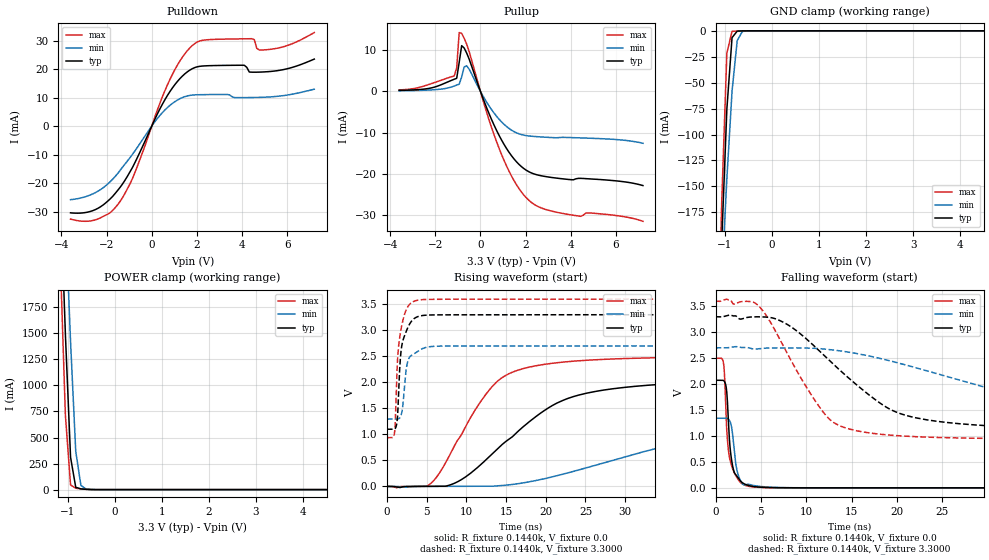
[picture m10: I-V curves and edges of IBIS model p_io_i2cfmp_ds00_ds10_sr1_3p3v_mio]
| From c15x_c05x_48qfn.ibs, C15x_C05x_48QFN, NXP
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[Model] p_io_i2cfmp_ds00_ds10_sr1_3p3v_mio
|   Model p_io_i2cfmp_ds00_ds10_sr1_3p3v_mio
| This model was characterised for following simulation conditions:
| External (pad) voltage:
|   - Typ: 3.3V,   - Min: 2.7V,   - Max: 3.6V
| Library cells for typ/min/max conditions are connected as defined below:
|  pad - External Pad
|  ipp_do_lv - Core Input
|  ipp_obe_lv - Output Buffer Enable
|  IOGC - NC
|  REFH3V3 - REFH3V3
|  REFL3V3 - REFL3V3
|  ZI - NC
|  abut_ncal_vddio[1] - vddio
|  abut_ncal_vddio[2] - vddio
|  abut_ncal_vddio[3] - vssio
|  abut_ncal_vddio[4] - vddio
|  abut_ncal_vddio[5] - vddio
|  abut_ncal_vddio[6] - vssio
|  abut_pcal_vddio[1] - vssio
|  abut_pcal_vddio[2] - vssio
|  abut_pcal_vddio[3] - vddio
|  abut_pcal_vddio[4] - vssio
|  abut_pcal_vddio[5] - vssio
|  abut_pcal_vddio[6] - vddio
|  ipp_do_1p8v - ipp_do_1p8v
|  ipp_dse_lv[0] - 0
|  ipp_dse_lv[1] - 0
|  ipp_eftd_lv - NC
|  ipp_ina_mux_vddio - NC
|  ipp_ina_mux_vddio[0] - NC
|  ipp_ina_mux_vddio[1] - NC
|  ipp_ina_r0_vddio - NC
|  ipp_ina_r0a_vddio - NC
|  ipp_ina_r0b_vddio - NC
|  ipp_ina_r0c_vddio - NC
|  ipp_ina_r0d_vddio - NC
|  ipp_ina_r0e_vddio - NC
|  ipp_ina_r0f_vddio - NC
|  ipp_ina_r300_vddio - NC
|  ipp_ina_r300a_vddio - NC
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Model_type I/O
Polarity   Non-Inverting
Enable   Active-High
Vinl =   0.9900V
Vinh =   2.3100V
Vmeas =  1.6500V
Cref =   30.0000pF
Rref =   1.0000M
Vref =   3.3000V
C_comp   1.7403pF   1.7015pF   1.7922pF
|C_comp_pullup   0.6955pF   0.7591pF   0.6584pF
|C_comp_pulldown   0.9315pF   0.9166pF   0.9304pF
[Model Spec]
| variable   typ   min   max
Vinh   2.3100V   1.8900V   2.5200V
Vinl   0.9900V   0.8100V   1.0800V
[Temperature Range]   25.0000   0.1250k   -40.0000
[Voltage Range]   3.3000V   2.7000V   3.6000V
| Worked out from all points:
|   slope of the pulldown table from 0 to 0.495 V, typ, clamps not added: 61.7 ohm
|   slope of the pullup table from 0 to 0.495 V, typ, clamps not added: 72.2 ohm
|   GND clamp passes 1 mA (typ) near -0.75 V on its own axis
|   POWER clamp passes 1 mA (typ) near -0.52 V on its own axis
|   rising waveform, R_fixture 0.1440k, V_fixture 0.0: 20-80 % time 10.5ns typ, 22.6ns min, 6.22ns max; typ from 0 V to 2.08 V
|   rising waveform, R_fixture 0.1440k, V_fixture 3.3000: 20-80 % time 727ps typ, 639ps min, 732ps max; typ from 1.1 V to 3.3 V
|   falling waveform, R_fixture 0.1440k, V_fixture 0.0: 20-80 % time 581ps typ, 619ps min, 625ps max; typ from 2.08 V to 0 V
|   falling waveform, R_fixture 0.1440k, V_fixture 3.3000: 20-80 % time 8.91ns typ, 19.6ns min, 5.37ns max; typ from 3.3 V to 1.1 V
[Pulldown]
|Voltage   I(typ)   I(min)   I(max)
-3.6V     -30.44mA   -25.83mA   -32.65mA
-2.39V    -28.88mA   -22.87mA   -32.61mA
-1.4V     -21.46mA   -15.51mA   -26.39mA
-850mV    -14.46mA   -9.856mA   -18.31mA
800mV     12.05mA    7.226mA    16.28mA
1.35V     17.48mA    9.968mA    24.09mA
1.9V      20.5mA     10.93mA    28.91mA
4.1V      21.31mA    9.981mA    30.6mA
4.43V     18.9mA     10mA       30.65mA
4.65V     18.9mA     10.03mA    27.3mA
5.09V     19.05mA    10.15mA    26.78mA
7.2V      23.49mA    12.93mA    32.8mA
[Pullup]
|Voltage   I(typ)   I(min)   I(max)
-3.6V     205.5uA    122.8uA    318.7uA
-1.16V    2.91mA     1.263mA    3.707mA
-1.05V    3.138mA    1.494mA    5.669mA
-940mV    6.993mA    1.733mA    14.21mA
-830mV    11.04mA    3.449mA    14mA
-720mV    10.47mA    5.872mA    12.85mA
-610mV    9.27mA     6.173mA    11.42mA
820mV     -10.6mA    -6.722mA   -13.7mA
1.48V     -16.32mA   -9.741mA   -21.54mA
2.03V     -19.11mA   -10.73mA   -25.77mA
3.46V     -21.08mA   -11.23mA   -29.38mA
7.2V      -22.83mA   -12.59mA   -31.48mA
[GND_clamp]
|Voltage   I(typ)   I(min)   I(max)
-3.6V     -4.377A    -3.283A    -5.855A
-1.18V    -351.7mA   -346.5mA   -367.9mA
-1.07V    -204.2mA   -241.2mA   -166.2mA
-960mV    -75.42mA   -142.6mA   -21.4mA
-850mV    -6.575mA   -58.21mA   -529.8uA
-740mV    -281.6uA   -9.383mA   -183.8uA
-630mV    -73.66uA   -605.1uA   -74.76uA
-410mV    -3.148uA   -9.219uA   -1.868uA
7.2V      0A         0A         0A
[POWER_clamp]
|Voltage   I(typ)   I(min)   I(max)
-3.6V     34.56A     31.8A      37.41A
-1.16V    2.902A     3.904A     2.233A
-1.05V    1.495A     2.658A     715.5mA
-940mV    310.6mA    1.419A     44.07mA
-830mV    22.38mA    368.3mA    13.28mA
-720mV    6.713mA    39.84mA    7.005mA
-610mV    2.702mA    5.591mA    2.612mA
7.2V      0A         0A         0A
[Ramp]
| variable   typ   min   max
dV/dt_r  1.2453/10.4856n   0.8037/22.6314n   1.5009/6.2179n
dV/dt_f  1.3210/8.9083n   0.8417/19.6092n   1.5979/5.3668n
R_load = 0.1440k
[Rising Waveform]
R_fixture= 0.1440k
V_fixture= 0.0
V_fixture_min= 0.0
V_fixture_max= 0.0
|time   V(typ)   V(min)   V(max)
0s        5.868nV    472.7nV    20.52nV
5.236ns   -163.4uV   -351.1uV   24.85mV
6.681ns   1.095mV    -73.88uV   272.9mV
8.765ns   78.63mV    -63.29uV   854.5mV
13.97ns   729.7mV    10.44mV    2.03V
20.87ns   1.559V     185.3mV    2.368V
30.4ns    1.911V     585.8mV    2.46V
41.3ns    2.011V     980.8mV    2.488V
51.9ns    2.047V     1.156V     2.497V
133.4ns   2.076V     1.339V     2.502V
[Rising Waveform]
R_fixture= 0.1440k
V_fixture= 3.3000
V_fixture_min= 2.7000
V_fixture_max= 3.6000
|time   V(typ)   V(min)   V(max)
0s        1.098V     1.293V     936.9mV
949.5ps   1.101V     1.293V     1.027V
1.046ns   1.114V     1.294V     1.229V
1.234ns   1.205V     1.293V     2.118V
1.376ns   1.459V     1.295V     2.536V
1.673ns   2.426V     1.333V     2.932V
2.007ns   2.802V     1.565V     3.192V
2.639ns   3.057V     2.412V     3.457V
4.081ns   3.273V     2.618V     3.585V
133.4ns   3.3V       2.7V       3.6V
[Falling Waveform]
R_fixture= 0.1440k
V_fixture= 0.0
V_fixture_min= 0.0
V_fixture_max= 0.0
|time   V(typ)   V(min)   V(max)
0s        2.076V     1.344V     2.502V
896.8ps   2.067V     1.343V     2.38V
1.004ns   2.045V     1.343V     2.111V
1.221ns   1.871V     1.342V     1.149V
1.601ns   774mV      1.277V     529.8mV
1.982ns   345.3mV    858.3mV    321.9mV
2.249ns   250.2mV    439.3mV    229.1mV
2.568ns   169.6mV    215mV      141.6mV
4.124ns   27.44mV    47.95mV    18.39mV
133.4ns   177.3nV    3.605uV    35.37nV
[Falling Waveform]
R_fixture= 0.1440k
V_fixture= 3.3000
V_fixture_min= 2.7000
V_fixture_max= 3.6000
|time   V(typ)   V(min)   V(max)
0s        3.3V       2.7V       3.6V
4.555ns   3.299V     2.679V     3.54V
7.828ns   3.16V      2.699V     2.619V
12.37ns   2.49V      2.67V      1.359V
17.79ns   1.679V     2.511V     1.042V
20.82ns   1.407V     2.378V     998.5mV
25.31ns   1.265V     2.158V     968.1mV
36.51ns   1.153V     1.655V     944.7mV
46.88ns   1.122V     1.469V     939.5mV
133.4ns   1.098V     1.297V     936.9mV
